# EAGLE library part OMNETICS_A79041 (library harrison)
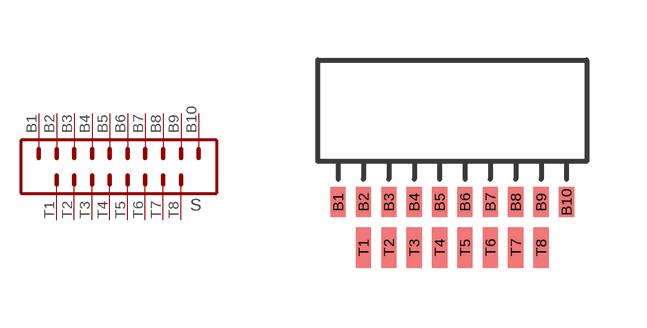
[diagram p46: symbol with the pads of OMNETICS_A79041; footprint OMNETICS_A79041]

Designator prefix S

## OMNETICS_A79041  [OMNETICS_A79041]
B1  B1  pas
B2  B2  pas
B3  B3  pas
B4  B4  pas
B5  B5  pas
B6  B6  pas
B7  B7  pas
B8  B8  pas
B9  B9  pas
B10  B10  pas
T1  T1  pas
T2  T2  pas
T3  T3  pas
T4  T4  pas
T5  T5  pas
T6  T6  pas
T7  T7  pas
T8  T8  pas

## Footprint OMNETICS_A79041 (pad centres in mm)
smd 0.381 x 0.762: B1 -2.857,-1.016; B2 -2.223,-1.016; B3 -1.587,-1.016; B4 -0.953,-1.016; B5 -0.318,-1.016; B6 0.318,-1.016; B7 0.953,-1.016; B8 1.587,-1.016; B9 2.223,-1.016; B10 2.857,-1.016
smd 0.381 x 1.016: T1 -2.223,-2.159; T2 -1.587,-2.159; T3 -0.953,-2.159; T4 -0.318,-2.159; T5 0.318,-2.159; T6 0.953,-2.159; T7 1.587,-2.159; T8 2.223,-2.159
